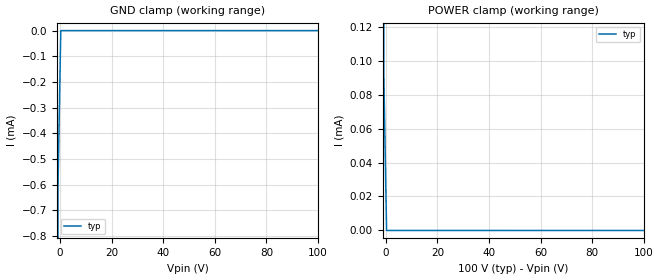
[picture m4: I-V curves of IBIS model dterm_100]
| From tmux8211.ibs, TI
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| dterm_100
[Model]   dterm_100
Model_type   Terminator
|   typ   min   max
C_comp   6.362683e-12   NA   NA
[Voltage Range]   100   NA   NA
[Temperature Range]   27   NA   NA
[Power Clamp Reference]   100   NA   NA
[GND Clamp Reference]   0   NA   NA
[GND Clamp]
|   Voltage   I(typ)   I(min)   I(max)
-5V       -1.446A    NA         NA
-1.818V   -221.6mA   NA         NA
-757.6mV  -598.9uA   NA         NA
303mV     -323.1pA   NA         NA
100V      2.552nA    NA         NA
[POWER Clamp]
|   Voltage   I(typ)   I(min)   I(max)
-5V       744mA      NA         NA
-1.818V   145.4mA    NA         NA
-758mV    90.5uA     NA         NA
303mV     2.547nA    NA         NA
100V      -327pA     NA         NA
